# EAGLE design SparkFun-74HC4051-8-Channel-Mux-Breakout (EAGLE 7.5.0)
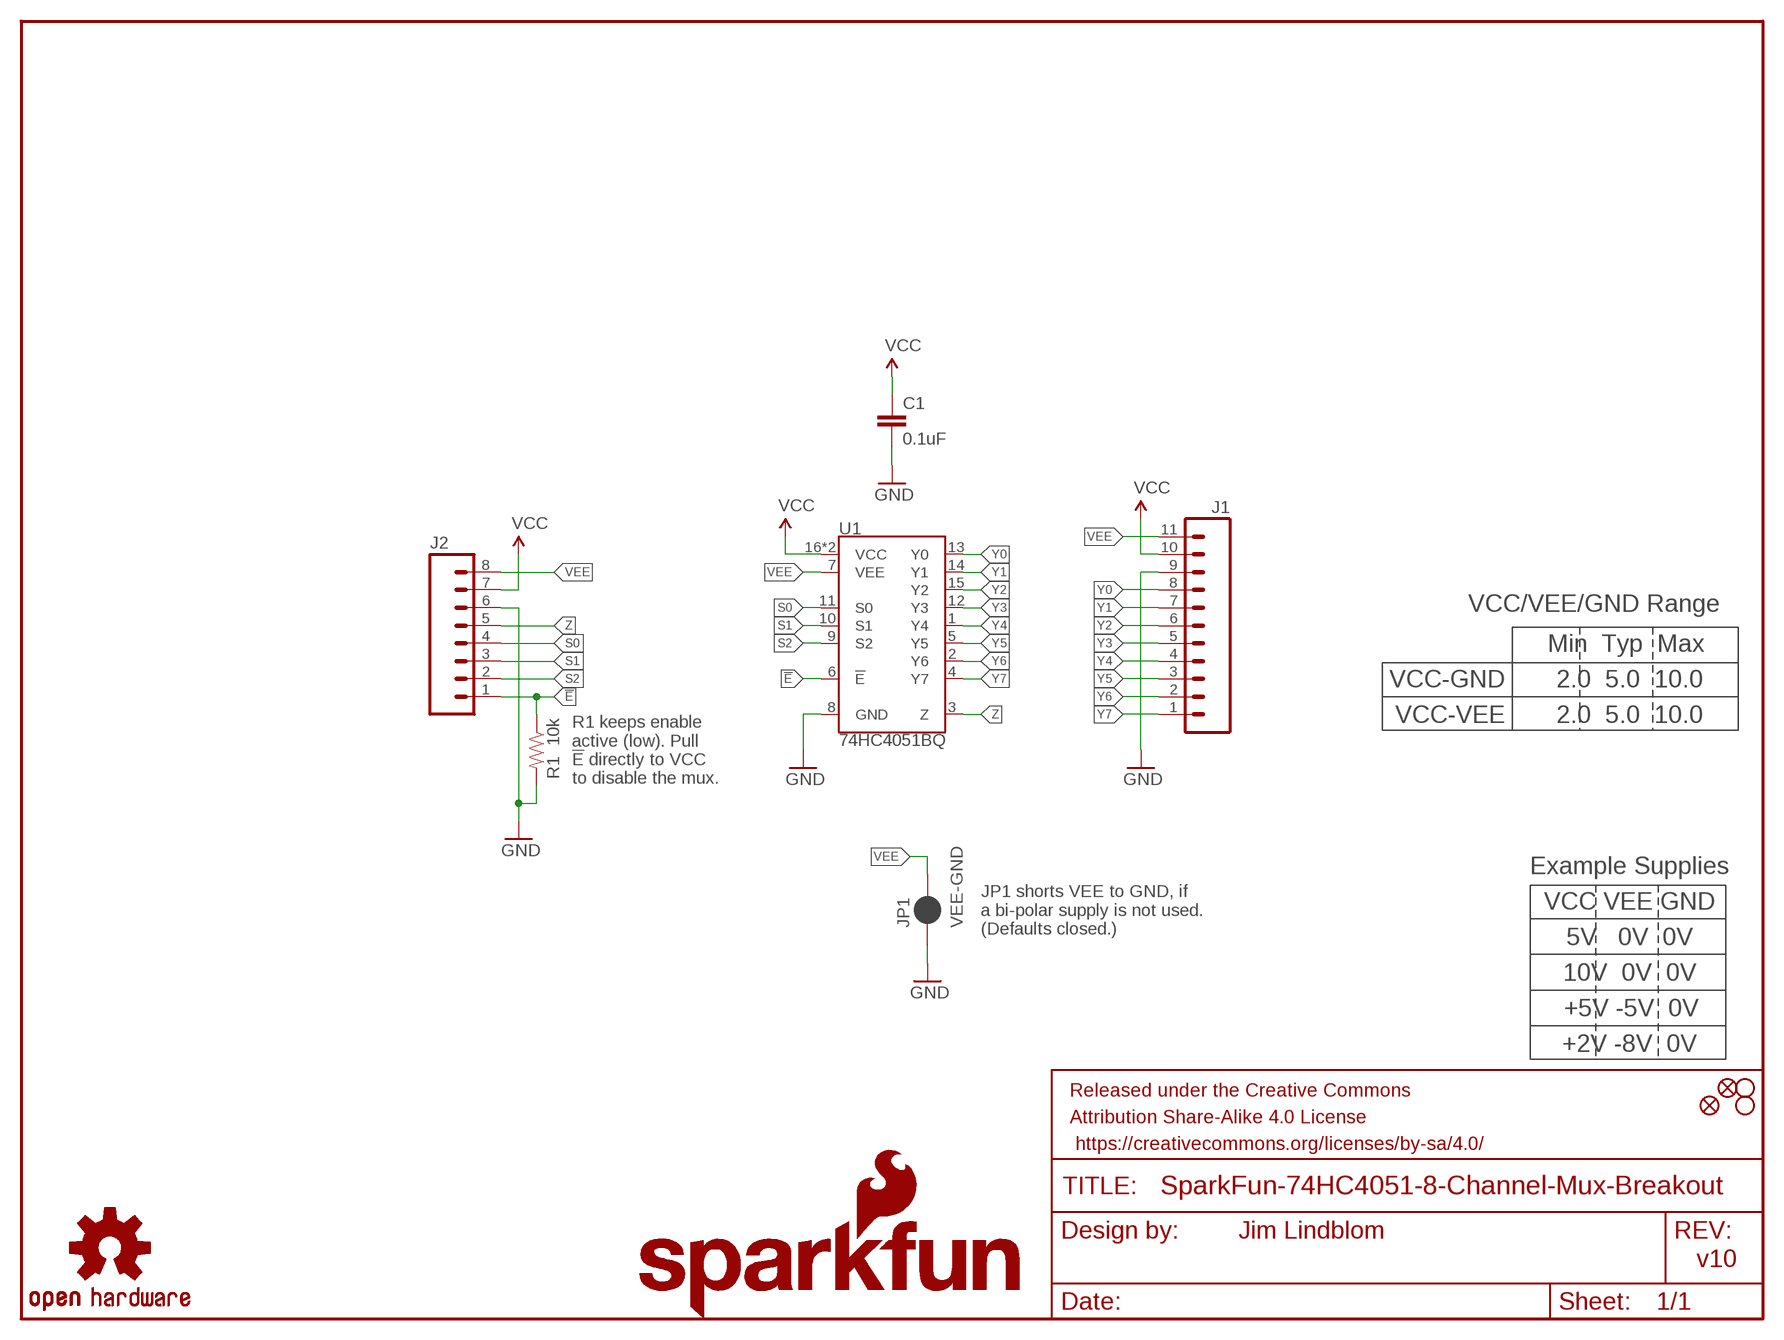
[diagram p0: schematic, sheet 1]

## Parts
C1  0.1uF  0.1UF-0603-25V-(+80/-20%)  [0603]
FD1  FIDUCIAL1X2  [FIDUCIAL-1X2]
FD2  FIDUCIAL1X2  [FIDUCIAL-1X2]
FRAME1  FRAME-LETTER  [CREATIVE_COMMONS]
H1  STAND-OFF  [STAND-OFF]
H2  STAND-OFF  [STAND-OFF]
J1  M11PTH  [1X11]
J2  M08  [1X08_ROUND]
JP1  VEE-GND  JUMPER-PAD-2-NC_BY_PASTENO-SILK  [PAD-JUMPER-2-NC_BY_PASTE_NO_SILK]
LOGO1  SFE_LOGO_FLAME.1_INCH  [SFE_LOGO_FLAME_.1]
LOGO2  OSHW-LOGOMINI  [OSHW-LOGO-MINI]
LOGO3  SFE_LOGO_NAME.1_INCH  [SFE_LOGO_NAME_.1]
R1  10k  10KOHM-0603-1/10W-1%  [0603]
U1  74HC4051BQ  [DHVQFN-16-2.5X3.5MM]

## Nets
!E!: J2.1 R1.1 U1.6(!E!)
GND: C1.2 J1.9 J2.6 JP1.1 R1.2 U1.8(GND)
S0: J2.4 U1.11(S0)
S1: J2.3 U1.10(S1)
S2: J2.2 U1.9(S2)
VCC: C1.1 J1.10 J2.7 U1.16(VCC) U1.EP(VCC)
VEE: J1.11 J2.8 JP1.2 U1.7(VEE)
Y0: J1.8 U1.13(Y0)
Y1: J1.7 U1.14(Y1)
Y2: J1.6 U1.15(Y2)
Y3: J1.5 U1.12(Y3)
Y4: J1.4 U1.1(Y4)
Y5: J1.3 U1.5(Y5)
Y6: J1.2 U1.2(Y6)
Y7: J1.1 U1.4(Y7)
Z: J2.5 U1.3(Z)

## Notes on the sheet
- VCC/VEE/GND Range
- Min  Typ  Max
- VCC-GND | 2.0  5.0  10.0
- VCC-VEE | 2.0  5.0  10.0
- R1 keeps enable 
  active (low). Pull 
  !E! directly to VCC 
  to disable the mux.
- Example Supplies
- VCC VEE GND
- JP1 shorts VEE to GND, if 
  a bi-polar supply is not used.
  (Defaults closed.)
- 5V   0V  0V
- 10V  0V  0V
- +5V -5V  0V
- +2V -8V  0V
- Jim Lindblom
- v10

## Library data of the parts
C1 = SparkFun-Capacitors:0.1UF: 0.1µF ceramic capacitors; PROD_ID: CAP-00810
FD1 FD2 = SparkFun-Aesthetics:FIDUCIAL: Fiducial Alignment Points
FRAME1 = SparkFun-Aesthetics:FRAME-LETTER: Schematic Frame
H1 H2 = SparkFun-Electromechanical:STAND-OFF: #4 Stand Off
J1 = SparkFun-Connectors:M11: Header 11 Standard 11-pin 0.1" header. Use with straight break away headers (SKU : PRT-00116), right angle break away headers (PRT-00553), swiss pins (PRT-00743), machine pins (PRT-00117), and female headers (PRT-00115).
J2 = SparkFun-Connectors:M08: Header 8 Standard 8-pin 0.1" header. Use with straight break away headers (SKU : PRT-00116), right angle break away headers (PRT-00553), swiss pins (PRT-00743), machine pins (PRT-00117), and female headers (PRT-00115).; PROD_ID: CONN-08437
JP1 = SparkFun-Passives:JUMPER-PAD-2-NC_BY_PASTE
LOGO1 = SparkFun-Aesthetics:SFE_LOGO_FLAME: SFE Logo, flame only
LOGO2 = SparkFun-Aesthetics:OSHW-LOGO: Open Source Hardware Logo
LOGO3 = SparkFun-Aesthetics:SFE_LOGO_NAME: SFE Logo, name only
R1 = SparkFun-Resistors:10KOHM: 10kΩ resistor; PROD_ID: RES-00824
U1 = 8mux:74HC4051: NXP 74HC4051 8-Channel Analog Multiplexer/Demultiplexer The 74HC4051; 74HCT4051 is a single-pole octal-throw analog switch (SP8T) suitable for use in analog or digital 8:1 multiplexer/demultiplexer applications. The switch features three digital select inputs (S0, S1 and S2), eight independent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; PROD_ID: IC-13334

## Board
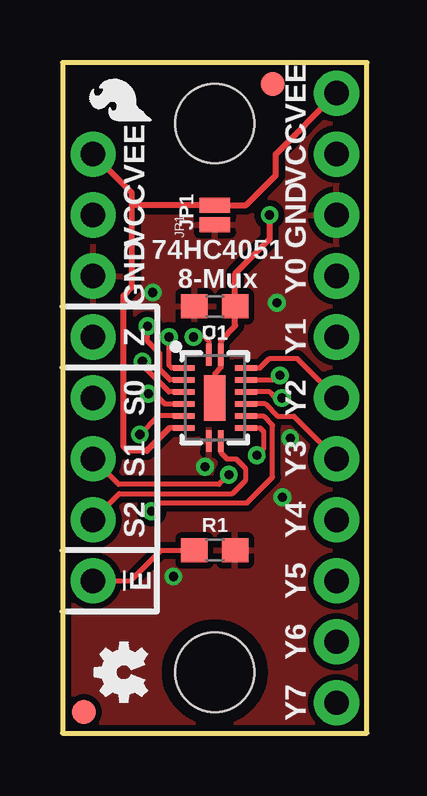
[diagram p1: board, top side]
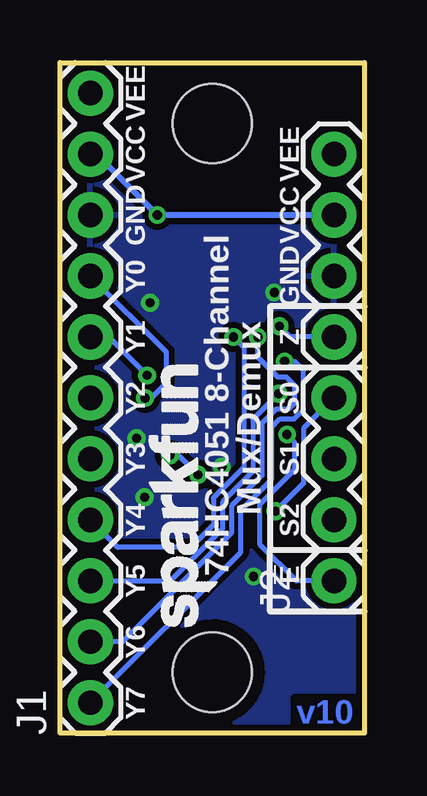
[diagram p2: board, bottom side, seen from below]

Size 12.7 x 27.94 mm. Coordinates in mm from the lower left corner, seen from the top.
Outline: 0,27.94 0,0 12.7,0 12.7,27.94 0,27.94
Copper layers (1*16): Top 0.035mm / dielectric 1.5mm / Bottom 0.035mm
Design rules "SparkFun-2-layer-TIGHT": minimum track width 7mil, minimum drill 15mil, track to track 7mil, track to pad 7mil, pad to pad 7mil, via to via 7mil, smd to smd 7mil, copper to edge 7mil, drill to drill 7mil, minimum pad ring 7mil, minimum via ring 7mil, stop-mask expansion 4mil, vias tented up to drill 25mil, thermal gap 10mil

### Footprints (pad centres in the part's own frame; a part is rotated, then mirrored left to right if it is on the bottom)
0603 = smd 1.1 x 1: 1 -0.85,0; 2 0.85,0
FIDUCIAL-1X2 = smd 1 x 1: 1 0,0
STAND-OFF = hole 3.302: 0,0
1X11 = drill 1.016 pad 1.88: 1 0,0; 2 2.54,0; 3 5.08,0; 4 7.62,0; 5 10.16,0; 6 12.7,0; 7 15.24,0; 8 17.78,0; 9 20.32,0; 10 22.86,0; 11 25.4,0
1X08_ROUND = drill 1.016 pad 1.88: 1 0,0; 2 2.54,0; 3 5.08,0; 4 7.62,0; 5 10.16,0; 6 12.7,0; 7 15.24,0; 8 17.78,0
PAD-JUMPER-2-NC_BY_PASTE_NO_SILK = smd 0.635 x 1.27: 1 -0.401,0; 2 0.413,0
DHVQFN-16-2.5X3.5MM = smd 0.9 x 0.24: 1 -1.8,-0.25; 8 1.8,-0.25; 9 1.8,0.25; 16 -1.8,0.25 | smd 0.24 x 0.9: 2 -1.25,-1.3; 3 -0.75,-1.3; 4 -0.25,-1.3; 5 0.25,-1.3; 6 0.75,-1.3; 7 1.25,-1.3; 10 1.25,1.3; 11 0.75,1.3; 12 0.25,1.3; 13 -0.25,1.3; 14 -0.75,1.3; 15 -1.25,1.3 | smd 1.9 x 0.9: EP 0,0

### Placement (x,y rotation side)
C1  6.35,17.78 180 top
FD1  0.89,0.89 0 top
FD2  8.76,27.05 0 top
FRAME1  not placed on the board
H1  6.35,25.4 0 top
H2  6.35,2.54 0 top
J1  11.43,1.27 90 bottom
J2  1.27,6.35 90 bottom
JP1  6.35,21.59 90 top
LOGO1  4.04,25.22 90 top
LOGO2  2.54,2.54 90 top
LOGO3  5.65,3.94 90 bottom
R1  6.35,7.62 0 top
U1  6.35,13.97 270 top

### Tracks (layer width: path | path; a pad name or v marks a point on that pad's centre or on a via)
!E!  (via drill 0.38)
  Top 0.203: U1.6 4,13.22 v3.23,12.45 | R1.1 4.12,7.62 2.85,6.35 J2.1
  Bottom 0.203: v3.23,12.45 2.92,12.14 2.92,10.97 4.37,9.53 4.37,7.87 2.85,6.35 J2.1
GND  (via drill 0.38)
  other vias: 9.5,12.29 3.76,18.36 8.94,17.93 5.94,11.1 9.17,9.83 4.62,6.53
  pour Top (isolate 0.254): 0,27.94 0,0 12.7,0 12.7,27.94
  pour Bottom (isolate 0.254): 12.7,27.94 12.7,0 0,0 0,27.94
S0  (via drill 0.38)
  Top 0.203: U1.11 8.37,13.22 8.76,12.83 8.76,10.67 7.7,9.6 4.06,9.6 v3.71,9.25
  Bottom 0.203: v3.71,9.25 2.54,10.41 2.54,12.7 J2.4
S1  (via drill 0.38)
  Top 0.203: U1.10 8.23,12.72 8.38,12.57 8.38,11.86 v8.1,11.58 | v6.93,10.77 6.53,10.36 2.34,10.36 J2.3
  Bottom 0.203: v8.1,11.58 7.75,11.58 v6.93,10.77
S2
  Top 0.203: U1.9 6.6,11.69 6.86,11.43 7.24,11.43 7.62,11.05 7.62,10.52 7.09,9.98 2.36,9.98 J2.2
VCC  (via drill 0.38)
  Top 0.203: U1.16
  Top 0.229: U1.EP 6.35,14.99 6.6,15.24 U1.16 | U1.16 6.6,16.38
  Top 0.254: 6.6,16.38 7.2,16.98 C1.1 7.2,19.14 8.64,20.57 v8.64,21.59
  Bottom 0.254: J1.10 11.18,24.13 v8.64,21.59 J2.7
VEE
  Top 0.229: U1.7 4.46,12.72
  Top 0.254: 2.9,22 2.9,18.59 2.54,18.24 2.54,11.94 2.72,11.76 3.5,11.76 4.46,12.72 | 2.9,22 2.9,22.5 J2.8 | 2.9,22 JP1.2 7.65,22 8.89,23.24 8.89,24.13 J1.11
Y0  (via drill 0.38)
  Top 0.203: v9.15,13.97 8.89,13.97 8.64,14.22 U1.13
  Bottom 0.203: v9.15,13.97 8.89,13.97 8.26,14.61 8.26,15.88 J1.8
Y1  (via drill 0.38)
  Top 0.203: U1.14 8.88,14.72 v9.07,14.91
  Bottom 0.203: v9.07,14.91 10.67,16.51 J1.7
Y2
  Top 0.203: U1.15 8.23,15.22 8.64,15.62 9.78,15.62 J1.6
Y3
  Top 0.203: U1.12 8.45,13.72 8.97,13.21 9.65,13.21 J1.5
Y4  (via drill 0.38)
  Top 0.203: v5.46,16.51 5.92,16.51 6.1,16.33 U1.1
  Bottom 0.203: v5.46,16.51 5.03,16.08 5.03,11.07 6.3,9.8 6.3,8.69 7.24,7.75 10.29,7.75 J1.4
Y5  (via drill 0.38)
  Top 0.203: v3.58,14.15 3.83,14.15 4.26,13.72 U1.5
  Bottom 0.203: v3.58,14.15 4.65,13.08 4.65,10.91 5.92,9.64 5.92,8.52 8.09,6.35 J1.3
Y6  (via drill 0.38)
  Top 0.203: v4.45,16.51 4.45,15.32 4.54,15.22 U1.2
  Bottom 0.203: v4.45,16.51 4.45,15.67 3.61,14.83 3.25,14.83 2.92,14.5 2.92,13.75 3.17,13.5 3.68,13.5 4.27,12.92 4.27,10.74 5.54,9.47 5.54,8.36 10.08,3.81 J1.2
Y7  (via drill 0.38)
  Top 0.203: v3.33,15.49 3.33,15.33 4.44,14.22 U1.4
  Bottom 0.203: v3.33,15.49 2.92,15.49 2.54,15.11 2.54,13.49 2.93,13.09 3.52,13.09 3.89,12.72 3.89,10.57 5.16,9.3 5.16,7.54 J1.1
Z  (via drill 0.38)
  Top 0.203: U1.3 4.48,14.72 4.06,15.14 4.06,15.81 3.54,16.33 v3.54,16.95
  Bottom 0.203: v3.54,16.95 3.1,16.51 J2.5

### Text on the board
Bottom: v10
tPlace: VEE | VEE | VCC | VCC | JP1 | GND | 74HC4051 / 8-Mux | GND | Y0 | Z | Y1 | S0 | Y2 | S1 | Y3 | S2 | Y4 | !E! | Y5 | Y6 | Y7
bPlace: VEE | VEE | VCC | VCC | GND | GND | Y0 | Z | Y1 | S0 | Y2 | S1 | Y3 | S2 | Mux/Demux | Y4 | !E! | 74HC4051 8-Channel | Y5 | Y6 | Y7
tDocu: Jim Lindblom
